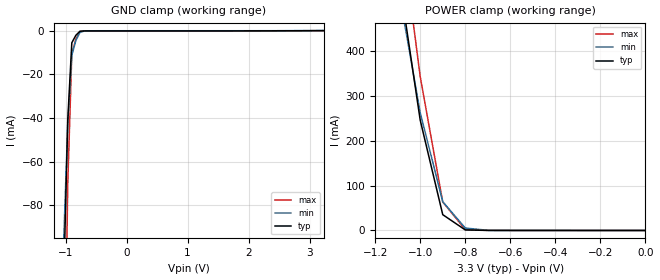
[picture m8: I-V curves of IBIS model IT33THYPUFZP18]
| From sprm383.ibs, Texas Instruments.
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|   Model Cell IT33THYPUFZP18
[Model]   IT33THYPUFZP18
Model_type   Input
Polarity   Non-Inverting
Vinl =  0.8V
Vinh =  2V
C_comp   0.5019789p   0.4562597p   0.5648978p
[Model Spec]
Vinl   0.8V   0.8V   0.8V
Vinh   2V   2V   2V
[Temperature Range]   25   105   0
[Voltage Range]   3.3   3.14   3.47
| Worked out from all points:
|   GND clamp passes 1 mA (typ) near -0.79 V on its own axis
|   POWER clamp passes 1 mA (typ) near -0.78 V on its own axis
[POWER_clamp]
|   voltage   I(typ)   I(min)   I(max)
-3.3V     9.936A     8.589A     10.91A
-1.067V   472.1mA    454mA      602.9mA
-1.033V   359.2mA    358.6mA    473.3mA
-1V       246.3mA    263.1mA    343.6mA
-900mV    35.32mA    64.33mA    63.62mA
-800mV    1.234mA    5.498mA    1.929mA
-700mV    130.3uA    388.1uA    162.6uA
-11.55fV  95.23nA    66.33nA    458.2nA
[GND_clamp]
|   voltage   I(typ)   I(min)   I(max)
-3.3V     -13.46A    -11.58A    -14.63A
-1.033V   -115.5mA   -96.35mA   -194.2mA
-966.7mV  -41.01mA   -42.91mA   -70.35mA
-900mV    -5.577mA   -11.26mA   -10.52mA
-833.3mV  -2.123mA   -4.53mA    -3.817mA
-766.7mV  -314.8uA   -866.4uA   -378.8uA
-700mV    -151.3uA   -264.4uA   -204.6uA
-500mV    -137.1uA   -72.34uA   -191.4uA
3.233V    -8.72uA    8.017uA    -38.34uA
